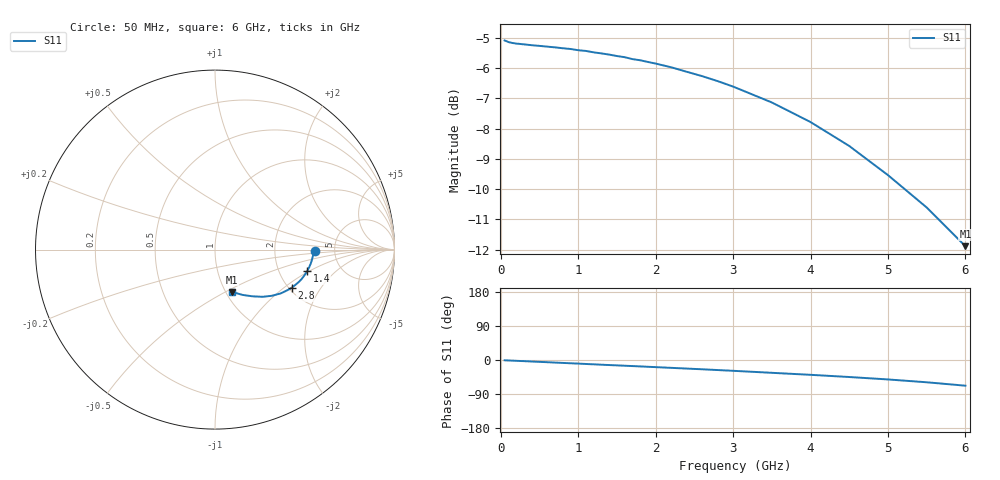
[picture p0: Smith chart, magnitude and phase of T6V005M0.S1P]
! SIEMENS Discrete & RF Semiconductors
! BAT62
! Si Schottky Diode in SOT143
! IF = 5 mA
! S-Parameters:  February  1997
# GHz  S  MA  R  50
!  f  S11
! GHz  MAG  ANG
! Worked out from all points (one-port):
!   34 points, 50 MHz to 6 GHz, reference 50 ohm
!   lowest |S11| = -11.9 dB at 6 GHz (marker M1), VSWR 1.68, Z = 53.6 - j27 ohm
!   |S11| at or under -10 dB: 5.217 GHz to end of sweep
!   S11 on the Smith chart (normalised r, x): 50 MHz: 3.50, -0.08; 1.4 GHz: 2.87, -0.96; 2.8 GHz: 2.07, -1.14; 6 GHz: 1.07, -0.54
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0.05  0.5561 -0.8
0.1  0.5527 -1.2
0.15  0.5508 -1.7
0.3  0.548 -3.0
0.4  0.5462 -4.0
0.6  0.5433 -5.8
0.7  0.5418 -6.8
0.8  0.54 -7.7
0.9  0.5384 -8.6
1  0.5359 -9.5
1.1  0.5344 -10.5
1.4  0.5271 -13.3
1.6  0.5219 -15.1
1.7  0.5181 -16.0
1.8  0.5159 -16.9
1.9  0.5126 -17.9
2  0.5094 -18.8
2.2  0.5023 -20.7
2.4  0.4939 -22.6
2.6  0.4857 -24.5
2.8  0.4767 -26.5
3  0.4668 -28.5
3.5  0.4395 -33.8
4  0.408 -39.1
4.5  0.3726 -44.9
5  0.3335 -51.3
5.5  0.295 -58.8
6  0.2547 -67.8
